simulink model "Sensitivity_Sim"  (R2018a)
settings: Solver=FixedStepAuto  StartTime=0.0  StopTime=80  FixedStep=Ts  MaxStep=0.000001  RelTol=1e-12  AbsTol=1e-8  EnableMultiTasking=on
InitFcn:
  | start
StopFcn:
  | pld
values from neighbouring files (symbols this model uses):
  Kq1 = I22*ww^2 - 3*wo2*(I11-I33)    [start.m]    (also in run.m)
  Kq2 = 2*I22*zet*ww    [start.m]    (also in run.m)
  Kqi = 0.0005    [start.m]    (also in run.m)
  Kr1 = (0.1*I11*I33*zet^2/Hy0) - sqrt( ((0.01^zet^4*I11^2*I33^2)/Hy0^2)+(4*I11*I33*zet^2) )    [start.m]    (also in run.m)
  Kr2 = 0.05*Kr1    [start.m]    (also in run.m)
  Kr3 = 0.04*zet*(Kr2-Hy0) * sqrt(abs(Hy0/(I11*I33)))    [start.m]    (also in run.m)
  Tmax = 0.05    [start.m]    (also in run.m)
  Ts = 0.01    [start.m]    (also in run.m = 0.001; runf.m = 0.0005)
undefined symbols (not defined in the file or in its folder): Avf, Bvf, Cvf, den, DiscIntNeverNeededParam, dsen, Dvf, nsen, num, RW_Steering
libraries: simulink x3

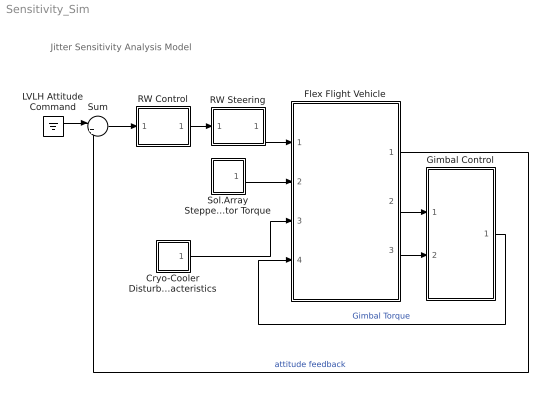
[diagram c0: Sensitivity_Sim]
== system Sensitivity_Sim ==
  note: Jitter Sensitivity Analysis Model
  Cryo-Cooler Disturbance Characteristics : Subsystem
  Flex Flight Vehicle : Subsystem
  Gimbal Control : Subsystem
  LVLH Attitude Command : Ground
  RW Control : Subsystem
  RW Steering : Subsystem
  Sol.Array Stepper-Motor Torque : Subsystem
  Sum : Sum  Inputs=|+-
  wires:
  Flex Flight Vehicle/2(alfa) -> Gimbal Control/1(Gimb)
  Flex Flight Vehicle/3(alfad) -> Gimbal Control/2(Grate)
  Sum/1 -> RW Control/1(atti)
  Flex Flight Vehicle/1(atti) -> Sum/2  "attitude feedback"
  RW Control/1(Tc) -> RW Steering/1(Trwc)
  RW Steering/1(Twi) -> Flex Flight Vehicle/1(Trw(i))
  Gimbal Control/1(GTrq) -> Flex Flight Vehicle/4(Tgimb)  "Gimbal Torque"
  LVLH Attitude Command/1 -> Sum/1
  Cryo-Cooler Disturbance Characteristics/1(Tdist) -> Flex Flight Vehicle/3(Tcryo)
  Sol.Array Stepper-Motor Torque/1(Tsa) -> Flex Flight Vehicle/2(Tsa)

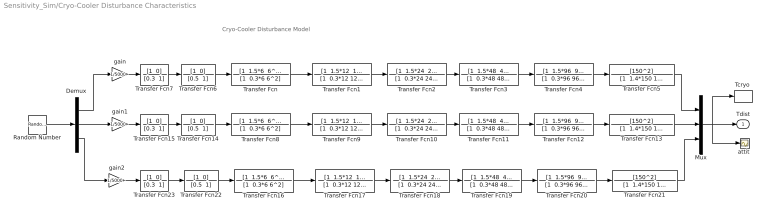
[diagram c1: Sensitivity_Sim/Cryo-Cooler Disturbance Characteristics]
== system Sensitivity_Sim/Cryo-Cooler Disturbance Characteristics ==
  note: Cryo-Cooler Disturbance Model
  Demux : Demux  Outputs=3
  Mux : Mux  Inputs=3
  Random Number : RandomNumber  Variance=[1 1 1]  Seed="[1  14  34]"  SampleTime=Ts
  "Tcryo " : ToWorkspace  VariableName=Tcryo  SampleTime=-1
  Transfer Fcn : TransferFcn  Numerator="[1  1.5*6  6^2]"  Denominator="[1  0.3*6 6^2]"
  Transfer Fcn1 : TransferFcn  Numerator="[1  1.5*12  12^2]"  Denominator="[1  0.3*12 12^2]"
  Transfer Fcn10 : TransferFcn  Numerator="[1  1.5*24  24^2]"  Denominator="[1  0.3*24 24^2]"
  Transfer Fcn11 : TransferFcn  Numerator="[1  1.5*48  48^2]"  Denominator="[1  0.3*48 48^2]"
  Transfer Fcn12 : TransferFcn  Numerator="[1  1.5*96  96^2]"  Denominator="[1  0.3*96 96^2]"
  Transfer Fcn13 : TransferFcn  Numerator=[150^2]  Denominator="[1  1.4*150 150^2]"
  Transfer Fcn14 : TransferFcn  Numerator="[1  0]"  Denominator="[0.5  1]"
  Transfer Fcn15 : TransferFcn  Numerator="[1  0]"  Denominator="[0.3  1]"
  Transfer Fcn16 : TransferFcn  Numerator="[1  1.5*6  6^2]"  Denominator="[1  0.3*6 6^2]"
  Transfer Fcn17 : TransferFcn  Numerator="[1  1.5*12  12^2]"  Denominator="[1  0.3*12 12^2]"
  Transfer Fcn18 : TransferFcn  Numerator="[1  1.5*24  24^2]"  Denominator="[1  0.3*24 24^2]"
  Transfer Fcn19 : TransferFcn  Numerator="[1  1.5*48  48^2]"  Denominator="[1  0.3*48 48^2]"
  Transfer Fcn2 : TransferFcn  Numerator="[1  1.5*24  24^2]"  Denominator="[1  0.3*24 24^2]"
  Transfer Fcn20 : TransferFcn  Numerator="[1  1.5*96  96^2]"  Denominator="[1  0.3*96 96^2]"
  Transfer Fcn21 : TransferFcn  Numerator=[150^2]  Denominator="[1  1.4*150 150^2]"
  Transfer Fcn22 : TransferFcn  Numerator="[1  0]"  Denominator="[0.5  1]"
  Transfer Fcn23 : TransferFcn  Numerator="[1  0]"  Denominator="[0.3  1]"
  Transfer Fcn3 : TransferFcn  Numerator="[1  1.5*48  48^2]"  Denominator="[1  0.3*48 48^2]"
  Transfer Fcn4 : TransferFcn  Numerator="[1  1.5*96  96^2]"  Denominator="[1  0.3*96 96^2]"
  Transfer Fcn5 : TransferFcn  Numerator=[150^2]  Denominator="[1  1.4*150 150^2]"
  Transfer Fcn6 : TransferFcn  Numerator="[1  0]"  Denominator="[0.5  1]"
  Transfer Fcn7 : TransferFcn  Numerator="[1  0]"  Denominator="[0.3  1]"
  Transfer Fcn8 : TransferFcn  Numerator="[1  1.5*6  6^2]"  Denominator="[1  0.3*6 6^2]"
  Transfer Fcn9 : TransferFcn  Numerator="[1  1.5*12  12^2]"  Denominator="[1  0.3*12 12^2]"
  "attit " : Scope
  gain : Gain  Gain=1/5000
  gain1 : Gain  Gain=1/5000
  gain2 : Gain  Gain=1/5000
  Tdist : Outport
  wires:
  Demux/1 -> gain/1
  Transfer Fcn/1 -> Transfer Fcn1/1
  Transfer Fcn1/1 -> Transfer Fcn2/1
  Transfer Fcn2/1 -> Transfer Fcn3/1
  Transfer Fcn3/1 -> Transfer Fcn4/1
  gain/1 -> Transfer Fcn7/1
  Transfer Fcn4/1 -> Transfer Fcn5/1
  Transfer Fcn5/1 -> Mux/1
  Transfer Fcn6/1 -> Transfer Fcn/1
  Transfer Fcn7/1 -> Transfer Fcn6/1
  Demux/2 -> gain1/1
  Transfer Fcn8/1 -> Transfer Fcn9/1
  Transfer Fcn9/1 -> Transfer Fcn10/1
  Transfer Fcn10/1 -> Transfer Fcn11/1
  Transfer Fcn11/1 -> Transfer Fcn12/1
  gain1/1 -> Transfer Fcn15/1
  Transfer Fcn12/1 -> Transfer Fcn13/1
  Transfer Fcn13/1 -> Mux/2
  Transfer Fcn14/1 -> Transfer Fcn8/1
  Transfer Fcn15/1 -> Transfer Fcn14/1
  Demux/3 -> gain2/1
  Transfer Fcn16/1 -> Transfer Fcn17/1
  Transfer Fcn17/1 -> Transfer Fcn18/1
  Transfer Fcn18/1 -> Transfer Fcn19/1
  Transfer Fcn19/1 -> Transfer Fcn20/1
  gain2/1 -> Transfer Fcn23/1
  Transfer Fcn20/1 -> Transfer Fcn21/1
  Transfer Fcn21/1 -> Mux/3
  Transfer Fcn22/1 -> Transfer Fcn16/1
  Transfer Fcn23/1 -> Transfer Fcn22/1
  Mux/1 -> Tdist/1, "attit "/1, "Tcryo "/1
  Random Number/1 -> Demux/1

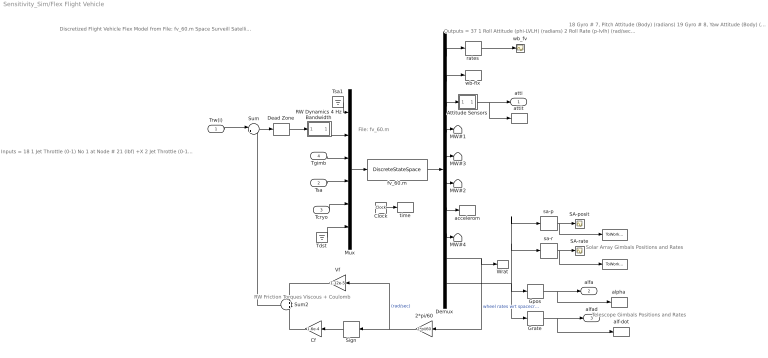
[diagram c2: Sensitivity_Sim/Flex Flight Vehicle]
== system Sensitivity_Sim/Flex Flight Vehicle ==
  note: Telescope Gimbals Positions and Rates
  note: Solar Array Gimbals Positions and Rates
  note: RW Friction Torques Viscous + Coulomb
  note: File: fv_60.m
  note: Outputs = 37 1 Roll Attitude (phi-LVLH) (radians) 2 Roll Rate (p-lvlh) (rad/sec) 3 Pitch Attitude (thet-LVLH) (radians) 4 Pitch Rate (q-lvlh) (rad/sec) 5 Yaw Attitude (psi-LVLH) (radians) 6 Yaw Rate (r-lvlh) (rad/sec) 7 Angle of attack, alfa, (radians) 8 Angle of sideslip, beta, (radian) 9 Change in Altitude, delta-h, (feet) 10 Forward Acceleration (V-dot) (ft/sec) 11 Cross Range Velocity (Vcr) (ft/sec) 12 Rate-Gyro # 1, Roll Rate (Body) (rad/sec) 13 Rate-Gyro # 2, Pitch Rate (Body) (rad/sec) 14 Rate-Gyro # 3, Yaw Rate (Body) (rad/sec) 15 Gyro # 4, Roll Attitude (Body) (radians) 16 Gyro # 5, Pitch Attitude (Body) (radians) 17 Gyro # 6, Yaw Attitude (Body) (radians)
  note: 18 Gyro # 7, Pitch Attitude (Body) (radians) 19 Gyro # 8, Yaw Attitude (Body) (radians) 20 Gyro # 9, Pitch Attitude (Body) (radians) 21 Gyro # 10, Yaw Attitude (Body) (radians) 22 Gyro # 11, Roll Attitude (Body) (radians) 23 Gyro # 12, Pitch Attitude (Body) (radians) 24 Gyro # 13, Yaw Attitude (Body) (radians) 25 Translat. Accelerom # 1, (along X), (ft/sec^2) 26 Translat. Accelerom # 2, (along Y), (ft/sec^2) 27 Reaction Wheel # 1 Rate (rpm) relative to vehicle 28 Reaction Wheel # 2 Rate (rpm) relative to vehicle 29 Reaction Wheel # 3 Rate (rpm) relative to vehicle 30 Rotation Angle at Elevati Gimbal No 1 31 Rotation Rate at Elevati Gimbal No 1 32 Rotation Angle at Azimuth Gimbal No 2 33 Rotation Rate at Azimuth Gimbal No 2 34 Rotation Angle at Rght SA Gimbal No 3 35 Rotation Rate at Rght SA Gimbal No 3 36 Rotation Angle at Left SA Gimbal No 4 37 Rotation Rate at Left SA Gimbal No 4
  note: Inputs = 18 1 Jet Throttle (0-1) No 1 at Node # 21 (lbf) +X 2 Jet Throttle (0-1) No 2 at Node # 22 (lbf) +X 3 Jet Throttle (0-1) No 3 at Node # 23 (lbf) +Y 4 Jet Throttle (0-1) No 4 at Node # 24 (lbf) -Y 5 Jet Throttle (0-1) No 5 at Node # 25 (lbf) -Y 6 Jet Throttle (0-1) No 6 at Node # 26 (lbf) +Y 7 Jet Throttle (0-1) No 7 at Node # 27 (lbf) +X 8 React-Wheel No 1 Torque to Spacecraft (ft-lb) 9 React-Wheel No 2 Torque to Spacecraft (ft-lb) 10 React-Wheel No 3 Torque to Spacecraft (ft-lb) 11 Elevation Trqu at Gimbal No 1 (ft-lb) 12 Azimuth Torque at Gimbal No 2 (ft-lb) 13 Rght SA Torque at Gimbal No 3 (ft-lb) 14 Left SA Torque at Gimbal No 4 (ft-lb) 15 Ext Torque Input 1 (ft-lb), dir: 1.00 0.00 0.00 16 Ext Torque Input 2 (ft-lb), dir: 0.00 1.00 0.00 17 Ext Torque Input 3 (ft-lb), dir: 0.00 0.00 1.00 18 Ext Torque Direct.=( 0.1970 -0.5964 -0.7782)
  note: Discretized Flight Vehicle Flex Model from File: fv_60.m Space Surveill Satellite with RCS and Reaction Wheels (Gimbals, 60 Modes, Z-Transf)
  Trw(i) : Inport
  Tsa : Inport  Port=2
  Tcryo : Inport  Port=3
  Tgimb : Inport  Port=4
  " " : ToWorkspace  VariableName=SA_pos  SampleTime=-1
  "   " : ToWorkspace  VariableName=SA_rate  SampleTime=-1
  2*pi/60 : Gain  Gain=2*pi/60
  Attitude Sensors : Subsystem
  Cf : Gain  Gain=1.6e-4
  Clock : Clock
  Dead Zone : DeadZone  LowerValue=-[1, 1]*Tmax/1000  UpperValue=[1 1]*Tmax/1000
  Demux : Demux  Outputs=[11, 3, 3, 2, 2, 3, 2, 1,2, 8]
  Gpos : Selector  InputPortWidth=8  IndexOptions=Index vector (dialog)  Indices=[1,3]  OutputSizes=1
  Grate : Selector  InputPortWidth=8  IndexOptions=Index vector (dialog)  Indices=[2, 4]  OutputSizes=1
  MW#{1..4} (4 alike) : Terminator
  Mux : Mux  Inputs=[7,3,2,2,3,1]
  RW Dynamics 4 Hz Bandwidth : Subsystem
  SA-posit : Scope
  SA-rate : Scope
  Sign : Signum
  Sum : Sum  Inputs=|+-
  Sum2 : Sum  Inputs=+|+
  Tdst : Ground
  Tsa1 : Ground
  Vf : Gain  Gain=1.12e-5
  Wrat : ToWorkspace  VariableName=wr  SampleTime=-1
  accelerom : ToWorkspace  VariableName=accel  SampleTime=-1
  alf-dot : ToWorkspace  VariableName=alfad  SampleTime=-1
  alpha : ToWorkspace  VariableName=alfa  SampleTime=-1
  attit : ToWorkspace  VariableName=atti  SampleTime=-1
  fv_60.m : DiscreteStateSpace  A=Avf  B=Bvf  C=Cvf  D=Dvf  SampleTime=Ts
  rates : Selector  InputPortWidth=11  IndexOptions=Index vector (dialog)  Indices=[2, 4, 6]  OutputSizes=1
  sa-p : Selector  InputPortWidth=8  IndexOptions=Index vector (dialog)  Indices=[5, 7]  OutputSizes=1
  sa-r : Selector  InputPortWidth=8  IndexOptions=Index vector (dialog)  Indices=[6, 8]  OutputSizes=1
  time : ToWorkspace  VariableName=time  SampleTime=-1
  wb-flx : ToWorkspace  VariableName=wb  SampleTime=-1
  wb_fv : Scope
  atti : Outport
  alfa : Outport  Port=2
  alfad : Outport  Port=3
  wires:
  Mux/1 -> fv_60.m/1
  Demux/9 -> 2*pi/60/1, Wrat/1  "wheel rates wrt spacecrft (rpm)"
  Demux/1 -> rates/1
  rates/1 -> wb_fv/1
  Demux/10 -> Gpos/1, Grate/1, sa-p/1, sa-r/1
  Demux/2 -> wb-flx/1
  Demux/7 -> accelerom/1
  Demux/3 -> Attitude Sensors/1(I)
  Grate/1 -> alfad/1, alf-dot/1
  Gpos/1 -> alfa/1, alpha/1
  Tsa/1 -> Mux/4
  Tdst/1 -> Mux/6
  Clock/1 -> time/1
  Tcryo/1 -> Mux/5
  sa-p/1 -> SA-posit/1, " "/1
  sa-r/1 -> SA-rate/1, "   "/1
  Vf/1 -> Sum2/1
  Cf/1 -> Sum2/2
  Sign/1 -> Cf/1
  2*pi/60/1 -> Sign/1, Vf/1  "(rad/sec)"
  Tgimb/1 -> Mux/3
  fv_60.m/1 -> Demux/1
  Trw(i)/1 -> Sum/1
  Sum/1 -> Dead Zone/1
  Sum2/1 -> Sum/2
  Dead Zone/1 -> RW Dynamics 4 Hz Bandwidth/1(I)
  RW Dynamics 4 Hz Bandwidth/1(O) -> Mux/2
  Attitude Sensors/1(O) -> atti/1, attit/1
  Tsa1/1 -> Mux/1
  Demux/6 -> MW#2/1
  Demux/5 -> MW#3/1
  Demux/4 -> MW#1/1
  Demux/8 -> MW#4/1

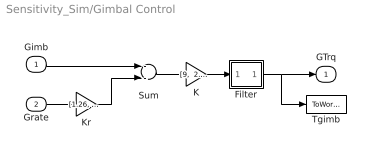
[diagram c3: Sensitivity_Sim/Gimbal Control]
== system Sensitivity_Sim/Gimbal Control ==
  Gimb : Inport
  Grate : Inport  Port=2
  Filter : Subsystem
  K : Gain  Gain="[9,  2.85]"
  Kr : Gain  Gain="[1.26,  1.14]"
  Sum : Sum  Inputs=--
  Tgimb : ToWorkspace  VariableName=Tgimb  SampleTime=-1
  GTrq : Outport
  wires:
  Sum/1 -> K/1
  Grate/1 -> Kr/1
  K/1 -> Filter/1(I)
  Filter/1(O) -> GTrq/1, Tgimb/1
  Gimb/1 -> Sum/1
  Kr/1 -> Sum/2

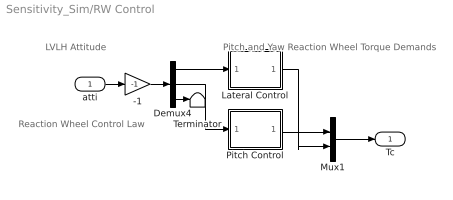
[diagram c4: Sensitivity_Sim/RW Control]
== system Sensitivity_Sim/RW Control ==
  note: Pitch and Yaw Reaction Wheel Torque Demands
  note: LVLH Attitude
  note: Reaction Wheel Control Law
  atti : Inport
  -1 : Gain  Gain=-1
  Demux4 : Demux  Outputs=3
  Lateral Control : Subsystem
  Mux1 : Mux  Inputs=2
  Pitch Control : Subsystem
  Terminator : Terminator
  Tc : Outport
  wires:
  Demux4/3 -> Terminator/1
  Demux4/1 -> Lateral Control/1(phi)
  Pitch Control/1(Tcy) -> Mux1/1
  Demux4/2 -> Pitch Control/1(the)
  atti/1 -> -1/1
  -1/1 -> Demux4/1
  Lateral Control/1(Tcz) -> Mux1/2
  Mux1/1 -> Tc/1

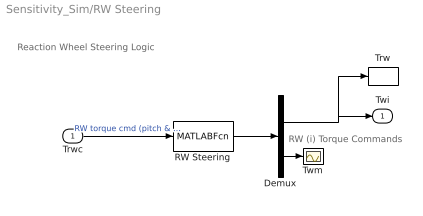
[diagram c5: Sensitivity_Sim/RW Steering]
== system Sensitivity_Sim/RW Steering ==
  note: RW (i) Torque Commands
  note: Reaction Wheel Steering Logic
  Trwc : Inport
  Demux : Demux  Outputs=[2, 1]
  RW Steering : MATLABFcn  MATLABFcn=RW_Steering( u(1:2) )  OutputDimensions=3
  Trw : ToWorkspace  VariableName=Trw  SampleTime=-1
  Twm : Scope
  Twi : Outport
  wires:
  Demux/1 -> Trw/1, Twi/1
  Trwc/1 -> RW Steering/1  "RW torque cmd (pitch & yaw)"
  RW Steering/1 -> Demux/1
  Demux/2 -> Twm/1

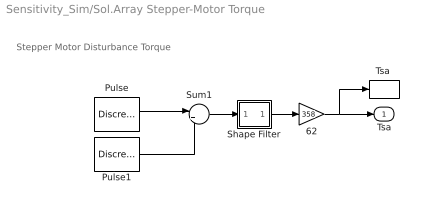
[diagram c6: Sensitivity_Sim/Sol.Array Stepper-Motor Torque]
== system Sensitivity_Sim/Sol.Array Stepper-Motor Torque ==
  note: Stepper Motor Disturbance Torque
  62 : Gain  Gain=358
  Pulse : DiscretePulseGenerator  PulseType=Time based  Amplitude="0.001*[1  1]"  Period="0.5*[1  1]"  PulseWidth="4*[1  1]"
  Pulse1 : DiscretePulseGenerator  PulseType=Time based  Amplitude="-0.001*[1  1]"  Period="0.5*[1  1]"  PulseWidth="4*[1  1]"  PhaseDelay="0.25*[1  1]"
  Shape Filter : Subsystem
  Sum1 : Sum  Inputs=|++
  "Tsa " : ToWorkspace  VariableName=Tsa  SampleTime=-1
  Tsa : Outport
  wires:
  Pulse/1 -> Sum1/1
  Pulse1/1 -> Sum1/2
  Sum1/1 -> Shape Filter/1(I)
  62/1 -> Tsa/1, "Tsa "/1
  Shape Filter/1(O) -> 62/1

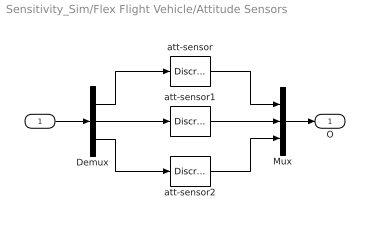
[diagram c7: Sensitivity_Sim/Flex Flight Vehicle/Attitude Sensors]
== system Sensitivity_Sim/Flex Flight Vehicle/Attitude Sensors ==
  I : Inport
  Demux : Demux  Outputs=3
  Mux : Mux  Inputs=3
  att-sensor : DiscreteTransferFcn  Numerator=[nsen]  Denominator=[dsen]  SampleTime=Ts
  att-sensor1 : DiscreteTransferFcn  Numerator=[nsen]  Denominator=[dsen]  SampleTime=Ts
  att-sensor2 : DiscreteTransferFcn  Numerator=[nsen]  Denominator=[dsen]  SampleTime=Ts
  O : Outport
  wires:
  I/1 -> Demux/1
  Mux/1 -> O/1
  att-sensor/1 -> Mux/1
  Demux/1 -> att-sensor/1
  Demux/3 -> att-sensor2/1
  att-sensor2/1 -> Mux/3
  Demux/2 -> att-sensor1/1
  att-sensor1/1 -> Mux/2

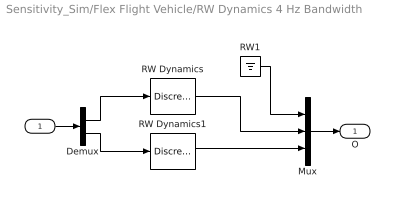
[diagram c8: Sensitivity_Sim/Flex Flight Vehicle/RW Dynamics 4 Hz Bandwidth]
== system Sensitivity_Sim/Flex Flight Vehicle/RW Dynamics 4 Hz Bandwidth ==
  I : Inport
  Demux : Demux  Outputs=2
  Mux : Mux  Inputs=3
  RW Dynamics : DiscreteTransferFcn  Numerator="[0  0.221199217]"  Denominator=[1 -0.778800783]  SampleTime=Ts
  RW Dynamics1 : DiscreteTransferFcn  Numerator="[0  0.221199217]"  Denominator=[1 -0.778800783]  SampleTime=Ts
  RW1 : Ground
  O : Outport
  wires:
  Demux/2 -> RW Dynamics1/1
  Demux/1 -> RW Dynamics/1
  RW Dynamics/1 -> Mux/2
  RW Dynamics1/1 -> Mux/3
  I/1 -> Demux/1
  Mux/1 -> O/1
  RW1/1 -> Mux/1

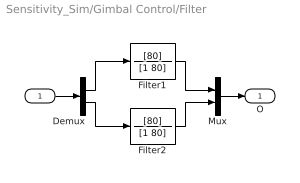
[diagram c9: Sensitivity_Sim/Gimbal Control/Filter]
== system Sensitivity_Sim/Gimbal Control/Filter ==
  I : Inport
  Demux : Demux  Outputs=2
  Filter1 : TransferFcn  Numerator=[80]  Denominator=[1 80]
  Filter2 : TransferFcn  Numerator=[80]  Denominator=[1 80]
  Mux : Mux  Inputs=2
  O : Outport
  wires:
  Mux/1 -> O/1
  I/1 -> Demux/1
  Demux/2 -> Filter2/1
  Demux/1 -> Filter1/1
  Filter2/1 -> Mux/2
  Filter1/1 -> Mux/1

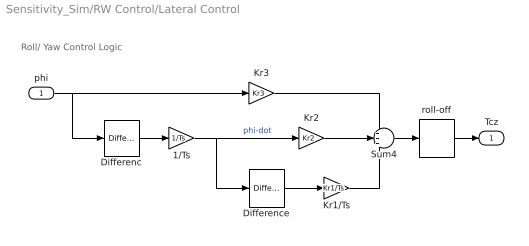
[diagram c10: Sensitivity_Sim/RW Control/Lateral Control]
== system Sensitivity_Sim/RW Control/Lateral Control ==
  note: Roll/ Yaw Control Logic
  phi : Inport
  1/Ts : Gain  Gain=1/Ts
  Differenc : simulink/Discrete/Difference  ICPrevInput=0.0  InputProcessing=Inherited  OutMin=[]  OutMax=[]  OutDataType=sfix(16)  OutScaling=2^-10  DoSatur=off
  Difference : simulink/Discrete/Difference  ICPrevInput=0.0  InputProcessing=Inherited  OutMin=[]  OutMax=[]  OutDataType=sfix(16)  OutScaling=2^-10  DoSatur=off
  Kr1/Ts : Gain  Gain=Kr1/Ts
  Kr2 : Gain  Gain=Kr2
  Kr3 : Gain  Gain=Kr3
  Sum4 : Sum  Inputs=+++
  roll-off : DiscreteTransferFcn  Numerator=[num]  Denominator=[den]  SampleTime=Ts
  Tcz : Outport
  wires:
  Kr3/1 -> Sum4/1
  Kr2/1 -> Sum4/2
  Kr1/Ts/1 -> Sum4/3
  phi/1 -> Kr3/1, Differenc/1
  Sum4/1 -> roll-off/1
  Difference/1 -> Kr1/Ts/1
  Differenc/1 -> 1/Ts/1
  1/Ts/1 -> Kr2/1, Difference/1  "phi-dot"
  roll-off/1 -> Tcz/1

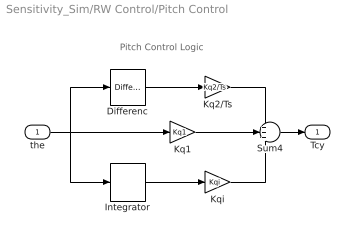
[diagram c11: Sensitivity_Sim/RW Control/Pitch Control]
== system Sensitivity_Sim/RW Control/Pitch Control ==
  note: Pitch Control Logic
  the : Inport
  Differenc : simulink/Discrete/Difference  ICPrevInput=0.0  InputProcessing=Inherited  OutMin=[]  OutMax=[]  OutDataType=sfix(16)  OutScaling=2^-10  DoSatur=off
  Integrator : DiscreteIntegrator  SampleTime=Ts  ICPrevOutput=DiscIntNeverNeededParam  ICPrevScaledInput=DiscIntNeverNeededParam
  Kq1 : Gain  Gain=Kq1
  Kq2/Ts : Gain  Gain=Kq2/Ts
  Kqi : Gain  Gain=Kqi
  Sum4 : Sum  Inputs=+++
  Tcy : Outport
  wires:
  Kq1/1 -> Sum4/2
  Sum4/1 -> Tcy/1
  Kq2/Ts/1 -> Sum4/1
  the/1 -> Kq1/1, Integrator/1, Differenc/1
  Kqi/1 -> Sum4/3
  Integrator/1 -> Kqi/1
  Differenc/1 -> Kq2/Ts/1

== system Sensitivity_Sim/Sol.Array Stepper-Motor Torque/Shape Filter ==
  I : Inport
  Demux : Demux  Outputs=2
  Mux : Mux  Inputs=2
  Transfer Fcn : TransferFcn  Numerator=[30^2]  Denominator="[1  2*30  30^2]"
  Transfer Fcn1 : TransferFcn  Numerator=[30^2]  Denominator="[1  2*30  30^2]"
  O : Outport
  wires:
  Demux/2 -> Transfer Fcn1/1
  Demux/1 -> Transfer Fcn/1
  Transfer Fcn/1 -> Mux/1
  Transfer Fcn1/1 -> Mux/2
  I/1 -> Demux/1
  Mux/1 -> O/1
